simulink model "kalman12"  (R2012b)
settings: Solver=ode45  StartTime=0.0  StopTime=100  RelTol=1e-3
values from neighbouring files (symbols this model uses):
  dtn = 0.01    [kalman_1.m]    (also in kalman_10.m; kalman_11.m; kalman_12.m; kalman_d1.m)
  Kest = kalman(P,1,0.01),    [LQG_1.m]    (also in ss_zwei_eing_1.m = kalman(sys2, Q, R))
  ki = -Kn(n+1)    [beobachter_2.m]    (also in beobachter_22.m; kalman_12.m = -Kn(3); kalman_13.m = -Kn(4); kalman_d1.m = -Kn(4))
  Kr = 2000    [aktiv_tilger_2.m]    (also in beobachter_22.m = 5; fuellstnd_3.m = 10,; fuellstnd_31.m = 10,; kalman_12.m = Kn(1:2))
  sys2 = sys1(:,[1,1,1])    [kalman_11.m]    (also in kalman_12.m; kalman_13.m = sys1(:,[1,1,1,1]); kalman_2.m = ss(H2); kalman_3.m = ss(H2))
  vnd = 1e-4    (= 0.0001)    [kalman_1.m]    (also in kalman_10.m; kalman_11.m; kalman_12.m; kalman_13.m = 0.01)
  vny = 1e-6    (= 1e-06)    [kalman_1.m]    (also in kalman_10.m; kalman_11.m = ', num2str(vny),' )']); kalman_12.m = ', num2str(vny),' )']); kalman_13.m = ', num2str(vny),' )']))
libraries: simulink x2

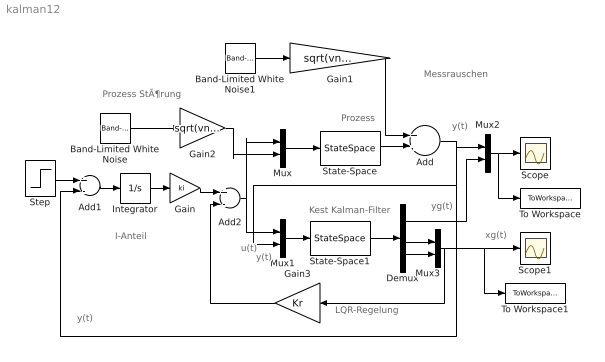
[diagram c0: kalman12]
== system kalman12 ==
  note: I-Anteil
  note: LQR-Regelung
  note: y(t)
  note: y(t)
  note: xg(t)
  note: u(t)
  note: y(t)
  note: yg(t)
  note: Messrauschen
  note: Prozess StÃ¶rung
  note: Kest Kalman-Filter
  note: Prozess
  Add : Sum
  Add1 : Sum  Inputs=+-
  Add2 : Sum  Inputs=+-
  Band-Limited White Noise : simulink/Sources/Band-Limited White Noise  Cov=[dtn, dtn]  Ts=dtn  seed=[23341, 2785]
  Band-Limited White Noise1 : simulink/Sources/Band-Limited White Noise  Cov=dtn  Ts=dtn  seed=[23341]
  Demux : Demux  Outputs=3
  Gain : Gain  Gain=ki
  Gain1 : Gain  Gain=sqrt(vny/dtn)
  Gain2 : Gain  Gain=sqrt(vnd/dtn)*eye(2,2)  Multiplication=Matrix(K*u)
  Gain3 : Gain  Gain=Kr  Multiplication=Matrix(K*u)
  Integrator : Integrator
  Mux{,1..3} (4 alike) : Mux  Inputs=2
  Scope : Scope
  Scope1 : Scope
  State-Space : StateSpace  A=sys2.a  B=sys2.b  C=sys2.c  D=sys2.d
  State-Space1 : StateSpace  A=Kest.a  B=Kest.b  C=Kest.c  D=Kest.d
  Step : Step  SampleTime=0
  To Workspace : ToWorkspace  VariableName=y  SampleTime=-1  SaveFormat=Structure With Time
  To Workspace1 : ToWorkspace  VariableName=y1  SampleTime=-1  SaveFormat=Structure With Time
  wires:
  Mux/1 -> State-Space/1
  Band-Limited White Noise/1 -> Gain2/1
  Gain2/1 -> Mux/2
  Band-Limited White Noise1/1 -> Gain1/1
  State-Space/1 -> Add/2
  Gain1/1 -> Add/1
  Add/1 -> Add1/2, Mux1/2, Mux2/1
  Mux1/1 -> State-Space1/1
  State-Space1/1 -> Demux/1
  Mux2/1 -> To Workspace/1, Scope/1
  Demux/1 -> Mux2/2
  Demux/2 -> Mux3/1
  Demux/3 -> Mux3/2
  Mux3/1 -> Gain3/1, To Workspace1/1, Scope1/1
  Step/1 -> Add1/1
  Add1/1 -> Integrator/1
  Integrator/1 -> Gain/1
  Gain/1 -> Add2/1
  Add2/1 -> Mux1/1, Mux/1
  Gain3/1 -> Add2/2
